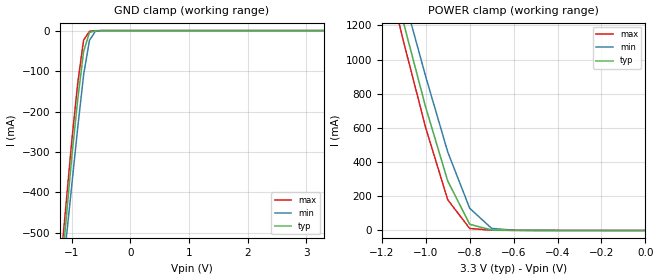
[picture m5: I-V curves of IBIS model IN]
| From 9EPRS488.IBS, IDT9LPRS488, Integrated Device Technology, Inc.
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|   Model IN
[Model]   IN
Model_type   Input
Polarity   Inverting
Vinl =   0.80V
Vinh =   2.00V
C_comp   3.40pF   2.85pF   3.95pF
[Temperature Range]   27.00   70.00   0.000
[Voltage Range]   3.30V   3.00V   3.70V
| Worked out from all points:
|   GND clamp passes 1 mA (typ) near -0.61 V on its own axis
|   POWER clamp passes 1 mA (typ) near -0.61 V on its own axis
[GND_clamp]
| voltage   I(typ)   I(min)   I(max)
-3.3V     -4.16A     -4.01A     -4.26A
-1.2V     -630mA     -670mA     -590mA
-1.1V     -470mA     -520mA     -430mA
-1V       -310mA     -380mA     -270mA
-900mV    -170mA     -240mA     -130mA
-800mV    -52.15mA   -110mA     -23.62mA
-700mV    -4.69mA    -24.32mA   -1.84mA
-600mV    -430uA     -1.9mA     -210uA
-500mV    -36.28uA   -150uA     -14.74uA
3.3V      150pA      24.16uA    -320pA
[POWER_clamp]
| voltage   I(typ)   I(min)   I(max)
-3.3V     13.35A     12.84A     13.68A
-1.2V     1.72A      1.85A      1.63A
-1.1V     1.21A      1.37A      1.1A
-1V       720mA      900mA      600mA
-900mV    290mA      460mA      180mA
-800mV    36.36mA    130mA      11.68mA
-700mV    2.84mA     12.08mA    1.52mA
-600mV    760uA      1.75mA     430uA
0V        150pA      200pA      170pA
